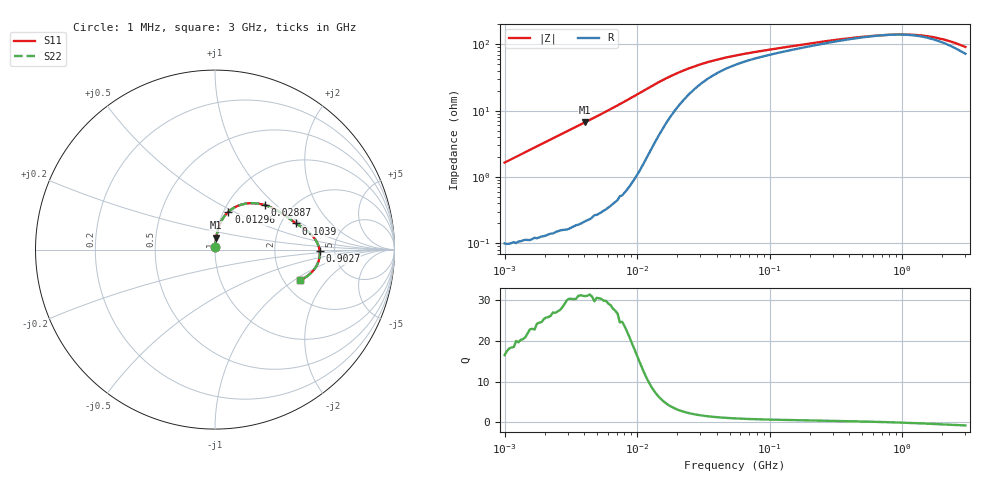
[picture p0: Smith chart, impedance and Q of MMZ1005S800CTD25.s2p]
! S-Parameter Data Generated by TDK Corporation
! Copyright(C) 2025 TDK Corporation.
! All Rights Reserved.
! TDK P/N: MMZ1005S800CTD25 (Chip Bead)
! Property: |Z|=80ohm at 100MHz
! Size(LxWxT): 1x0.5x0.5mm
! Model Type: s2p (Touchstone File Format Version 1.0)
! Frequency: DC=Yes Start=1MHz Stop=3000MHz 202points Log-sweep
! Model Generated on Feb. 6, 2025
! Terms and conditions regarding TDK Simulation Models:
! 1)This simulation model is being provided solely for informational
!  purposes. Please refer to the specifications of the products in
!  terms of detailed characteristics of such products.
! 2)In no event shall TDK Corporation of any of its subsidiaries be
!  liable for any loss or damage arising, directly or indirectly,
!  from any information contained in this simulation model, including,
!  but not limited to loss or damages arising from any inaccuracies,
!  omissions or errors in connection with such information.
! 3)Any and all copyrights on this simulation model are owned by
!  TDK Corporation.  Duplication or redistribution of this simulation
!  model without prior written permission from TDK Corporation
!  is prohibited.
! 4)This simulation model is subject to any modification or change
!  without any prior notice.
! 5)Neither TDK Corporation nor any of its subsidiaries shall make any
!  warranty, express or implied, including but not limited to the
!  correctness, implied warranties of merchantability and fitness for
!  a particular purpose with respect to this simulation models.
! 6)The use of this simulation model shall be deemed to have consented
!  to the terms and conditions hereof.
! Port Assignments:
!  1 ---@@@--- 2
! Applicable Conditions:
!  Temperature = 25 degC
!  DC Bias Current = 0 A
!  Small Signal Operation
# Hz S MA R 50
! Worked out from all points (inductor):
!   201 points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, 1 MHz to 3 GHz, reference 50 ohm
!   read as one part in series: L = 262 nH near 1.041 MHz
!   highest Q = 31.1 at 4.06 MHz (marker M1), where L = 262 nH
!   self-resonance near 833.4 MHz
!   S11 on the Smith chart (normalised r, x): 1 MHz: 1.00, +0.03; 12.96 MHz: 1.06, +0.47; 28.87 MHz: 1.47, +0.85; 103.9 MHz: 2.41, +0.91; 902.7 MHz: 3.80, -0.10; 3 GHz: 2.44, -1.12
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1000000  0.01646 85.6  0.9989 -0.9  0.9989 -0.9  0.01646 85.6
2139570  0.03509 85.8  0.998 -2.0  0.998 -2.0  0.03509 85.8
3900413  0.06394 84.5  0.9959 -3.7  0.9959 -3.7  0.06394 84.5
4059721  0.06651 84.3  0.9956 -3.8  0.9956 -3.8  0.06651 84.3
6058321  0.1001 82.3  0.9916 -5.7  0.9916 -5.7  0.1001 82.3
8345207  0.1403 79.4  0.9839 -8.1  0.9839 -8.1  0.1403 79.4
1.061086e7  0.1821 75.5  0.9706 -10.5  0.9706 -10.5  0.1821 75.5
1.29622e7  0.2239 70.4  0.9486 -12.8  0.9486 -12.8  0.2239 70.4
1.461624e7  0.2504 66.5  0.9291 -14.3  0.9291 -14.3  0.2504 66.5
1.934349e7  0.3082 56.2  0.8675 -17.2  0.8675 -17.2  0.3082 56.2
2.886629e7  0.3713 42.0  0.7656 -18.9  0.7656 -18.9  0.3713 42.0
3.820236e7  0.4023 34.0  0.7034 -18.6  0.7034 -18.6  0.4023 34.0
5.477226e7  0.4326 26.3  0.6417 -17.4  0.6417 -17.4  0.4326 26.3
1.039275e8  0.4755 17.9  0.5665 -14.9  0.5665 -14.9  0.4755 17.9
2.136344e8  0.5225 11.7  0.4997 -12.2  0.4997 -12.2  0.5225 11.7
4.219165e8  0.559 6.3  0.4485 -7.8  0.4485 -7.8  0.559 6.3
8.005644e8  0.5812 0.4  0.4188 -0.6  0.4188 -0.6  0.5812 0.4
9.0272e8  0.5833 -0.9  0.4169 1.2  0.4169 1.2  0.5833 -0.9
1.243477e9  0.5833 -4.8  0.4216 6.7  0.4216 6.7  0.5833 -4.8
1.712864e9  0.5711 -9.5  0.4469 12.2  0.4469 12.2  0.5711 -9.5
2.266846e9  0.5466 -14.3  0.4894 16.0  0.4894 16.0  0.5466 -14.3
3e9  0.5034 -19.8  0.5534 18.0  0.5534 18.0  0.5034 -19.8
